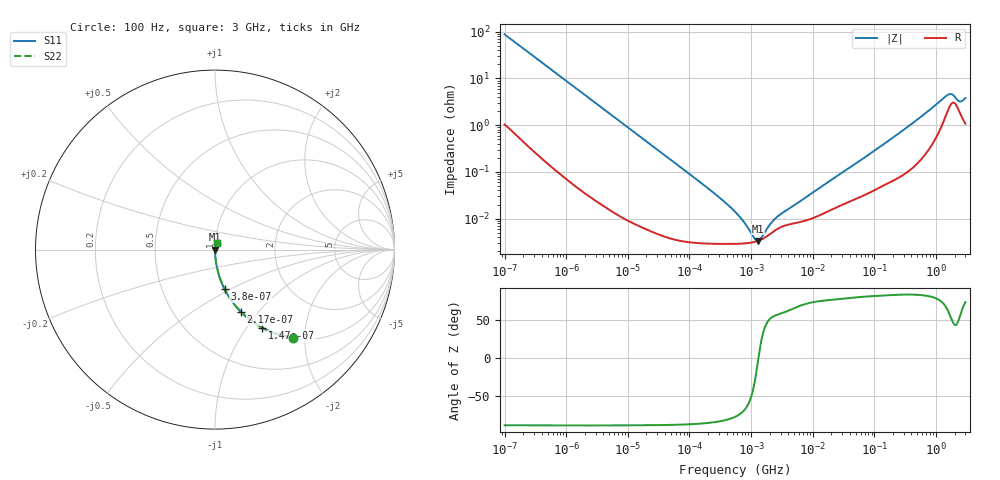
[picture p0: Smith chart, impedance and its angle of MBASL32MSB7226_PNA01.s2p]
! MBASL32MSB7226_PNA01  S-PARAMETER MODEL  ( Standard Model )
! Model Generated by TAIYO YUDEN Corporation (http://www.ty-top.com)
! Version 1.0
! TAIYO YUDEN Control No. 220601
! Copyright(c) 2015 TAIYO YUDEN CO.,LTD. All Rights Reserved.
! Product Description (link to TY-COMPAS)
! https://ds.yuden.co.jp/TYCOMPAS/or/detail?pn=MBASL32MSB7226KPNA01&u=M
! Products Name : Multilayer Ceramic Capacitors
! Characteristics :
!  Capacitance : 22 [uF] , Rated Voltage : 10 [V] , TCC : X7R
!  Case Size : 3.2 x 2.5 / 0.126 x 0.098 [mm/inch] , Thickness : 2.5 / 0.098 [mm/inch]
!  (Conditions: Temperature = 25 [degC] , DC Bias Voltage = 0 [V])
! External Node Assignments :
!  1  o---| |---o  2
! GND o---------o GND
! Frequency Range : 100Hz  -  3GHz  [ 401 STEP ]
# MHZ S RI R 50
! Freq[MHz].  S11 Real  S11 Imag  S21 Real  S21 Imag  S12 Real  S12 Imag  S22 Real  S22 Imag
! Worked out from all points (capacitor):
!   401 points, 100 Hz to 3 GHz, reference 50 ohm
!   read as one part in series: C = 18.1 uF near 109 Hz
!   lowest |Z| = 3.33 mohm at 1.295 MHz (marker M1)
!   series resonance near 1.316 MHz, so ESL is about 810 pH
!   S11 on the Smith chart (normalised r, x): 100 Hz: 1.02, -1.75; 147 Hz: 1.01, -1.19; 217 Hz: 1.01, -0.81; 380 Hz: 1.00, -0.47; 3 GHz: 1.02, +0.07
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0.0001  0.4347 -0.4898  0.5653 0.4898  0.5653 0.4898  0.4347 -0.4898
0.000147  0.2646 -0.4357  0.7354 0.4357  0.7354 0.4357  0.2646 -0.4357
0.000217  0.1439 -0.3461  0.8561 0.3461  0.8561 0.3461  0.1439 -0.3461
0.00038  0.0531 -0.2198  0.9469 0.2198  0.9469 0.2198  0.0531 -0.2198
0.000789  0.0133 -0.1107  0.9867 0.1107  0.9867 0.1107  0.0133 -0.1107
0.001788  0.00285 -0.0496  0.9971 0.0496  0.9971 0.0496  0.00285 -0.0496
0.005476  0.000409 -0.0163  0.9996 0.0163  0.9996 0.0163  0.000409 -0.0163
0.031977  5.33e-05 -0.00282  0.9999 0.00282  0.9999 0.00282  5.33e-05 -0.00282
0.231582  2.91e-05 -0.000379  1 0.000379  1 0.000379  2.91e-05 -0.000379
0.388167  2.87e-05 -0.000214  1 0.000214  1 0.000214  2.87e-05 -0.000214
0.547723  2.88e-05 -0.000138  1 0.000138  1 0.000138  2.88e-05 -0.000138
0.650627  2.9e-05 -0.000106  1 0.000106  1 0.000106  2.9e-05 -0.000106
0.740304  2.92e-05 -8.45e-05  1 8.45e-05  1 8.45e-05  2.92e-05 -8.45e-05
1.295438  3.32e-05 -2.18e-06  1 2.18e-06  1 2.18e-06  3.32e-05 -2.18e-06
2.470636  5.61e-05 8.33e-05  0.9999 -8.33e-05  0.9999 -8.33e-05  5.61e-05 8.33e-05
9.794414  0.000101 0.000339  0.9999 -0.000339  0.9999 -0.000339  0.000101 0.000339
175.1444  0.00061 0.00473  0.9994 -0.00473  0.9994 -0.00473  0.00061 0.00473
536.3016  0.00187 0.0141  0.9981 -0.0141  0.9981 -0.0141  0.00187 0.0141
1506.733  0.0195 0.0379  0.9805 -0.0379  0.9805 -0.0379  0.0195 0.0379
1789.813  0.0295 0.0339  0.9705 -0.0339  0.9705 -0.0339  0.0295 0.0339
2419.119  0.0193 0.025  0.9807 -0.025  0.9807 -0.025  0.0193 0.025
3000  0.0119 0.0357  0.9881 -0.0357  0.9881 -0.0357  0.0119 0.0357
